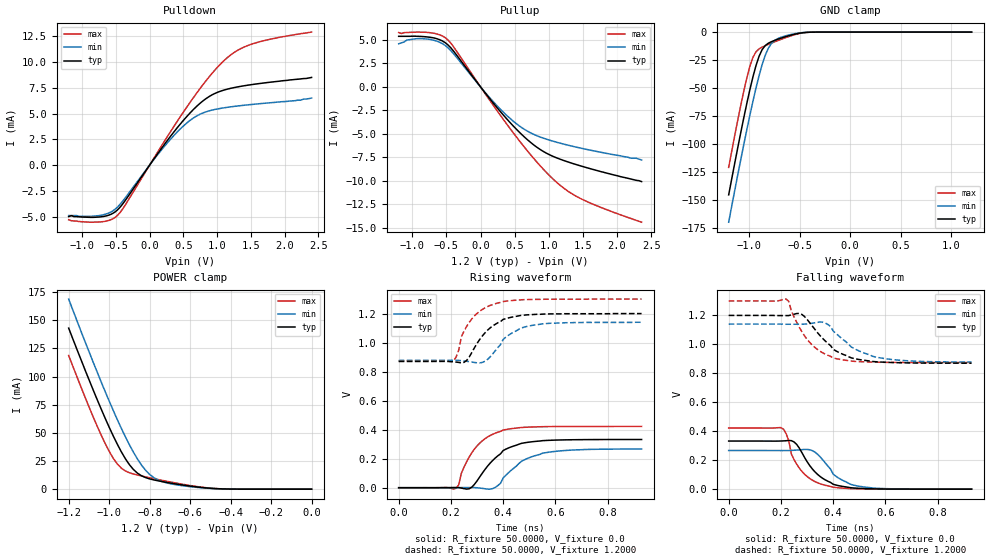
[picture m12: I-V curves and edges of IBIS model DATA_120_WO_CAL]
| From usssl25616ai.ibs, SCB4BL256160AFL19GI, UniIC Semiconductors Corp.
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|   Model DATA_120_WO_CAL
[Model]  DATA_120_WO_CAL
Model_type I/O
Polarity   Non-Inverting
Enable   Active-High
Vinl =   0.3800V
Vinh =   0.8200V
Vmeas =  0.6000V
Cref =   5.0000pF
Rref =   50.0000
Vref =   0.6000V
C_comp   1.7430pF   1.7110pF   1.7640pF
[Temperature Range]   25.0000   85.0000   -40.0000
[Voltage Range]   1.2000V   1.1400V   1.3000V
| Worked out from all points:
|   slope of the pulldown table from 0 to 0.18 V, typ, clamps not added: 108 ohm
|   slope of the pullup table from 0 to 0.18 V, typ, clamps not added: 108 ohm
|   GND clamp passes 1 mA (typ) near -0.50 V on its own axis
|   POWER clamp passes 1 mA (typ) near -0.51 V on its own axis
|   rising waveform, R_fixture 50.0000, V_fixture 0.0: 20-80 % time 103ps typ, 114ps min, 92.6ps max; typ from 0 V to 0.332 V
|   rising waveform, R_fixture 50.0000, V_fixture 1.2000: 20-80 % time 96ps typ, 92.4ps min, 78.1ps max; typ from 0.87 V to 1.2 V
|   falling waveform, R_fixture 50.0000, V_fixture 0.0: 20-80 % time 91.6ps typ, 90.4ps min, 73.1ps max; typ from 0.332 V to 0 V
|   falling waveform, R_fixture 50.0000, V_fixture 1.2000: 20-80 % time 115ps typ, 132ps min, 100ps max; typ from 1.2 V to 0.87 V
[Pulldown]
|Voltage   I(typ)   I(min)   I(max)
-1.2V     -5mA       -4.9mA     -5.3mA
-720mV    -5.02mA    -4.87mA    -5.507mA
-480mV    -4.371mA   -4.101mA   -4.906mA
-360mV    -3.417mA   -3.167mA   -3.855mA
200mV     1.839mA    1.668mA    2.116mA
520mV     4.485mA    3.908mA    5.332mA
680mV     5.593mA    4.698mA    6.829mA
840mV     6.469mA    5.177mA    8.219mA
1.2V      7.443mA    5.647mA    10.68mA
1.36V     7.649mA    5.774mA    11.33mA
1.6V      7.886mA    5.935mA    11.91mA
2.4V      8.5mA      6.5mA      12.9mA
[Pullup]
|Voltage   I(typ)   I(min)   I(max)
-1.2V     5.4mA      4.6mA      5.8mA
-1.08V    5.4mA      5mA        5.8mA
-880mV    5.39mA     5.16mA     5.84mA
-680mV    5.219mA    4.968mA    5.719mA
-520mV    4.73mA     4.433mA    5.263mA
-400mV    3.86mA     3.579mA    4.326mA
120mV     -1.12mA    -1.031mA   -1.272mA
440mV     -3.861mA   -3.41mA    -4.516mA
760mV     -6.076mA   -4.996mA   -7.465mA
1.08V     -7.464mA   -5.827mA   -9.945mA
1.48V     -8.455mA   -6.548mA   -11.96mA
2.36V     -10.1mA    -7.8mA     -14.43mA
[GND_clamp]
|Voltage   I(typ)   I(min)   I(max)
-1.2V     -145.3mA   -169.7mA   -120.8mA
-1.11V    -103.1mA   -127.3mA   -78.51mA
-1.05V    -76.2mA    -100.1mA   -52.43mA
-990mV    -51.2mA    -74mA      -30.39mA
-960mV    -39.9mA    -61.63mA   -22.48mA
-900mV    -21.67mA   -39mA      -15mA
-870mV    -15.78mA   -29.25mA   -13.45mA
-810mV    -10.04mA   -14.72mA   -11.07mA
-750mV    -7.557mA   -7.71mA    -8.865mA
-600mV    -3.111mA   -2.463mA   -3.804mA
-420mV    -215.4uA   -156.1uA   -235uA
1.2V      1.597nA    5.589nA    1.463nA
[POWER_clamp]
|Voltage   I(typ)   I(min)   I(max)
-1.2V     143mA      168.8mA    118.7mA
-1.06V    79.88mA    104.3mA    56.26mA
-1.02V    63.08mA    86.79mA    40.63mA
-980mV    47.32mA    69.97mA    27.48mA
-940mV    33.2mA     54.05mA    18.67mA
-880mV    17.43mA    32.78mA    13.45mA
-840mV    11.87mA    21.34mA    11.69mA
-800mV    9.133mA    13.1mA     10.12mA
-720mV    6.135mA    5.731mA    7.166mA
-560mV    1.838mA    1.456mA    2.161mA
-420mV    156.9uA    132.7uA    153uA
0V        1.597nA    1.927nA    2.16nA
[Ramp]
| variable   typ   min   max
dV/dt_r  0.1993/0.1052n   0.1601/0.1184n   0.2534/87.6937p
dV/dt_f  0.1979/0.1159n   0.1573/0.1322n   0.2551/93.0126p
R_load = 50.0000
[Rising Waveform]
R_fixture= 50.0000
V_fixture= 0.0
V_fixture_min= 0.0
V_fixture_max= 0.0
|time   V(typ)   V(min)   V(max)
0s        0V         0V         0V
220ps     1.212mV    191.5uV    -3.906mV
230ps     1.159mV    343uV      20.28mV
250ps     -6.397mV   813.1uV    141mV
290ps     22.9mV     785.4uV    266mV
360ps     188.1mV    -6.369mV   368.4mV
400ps     256.1mV    66.95mV    397.2mV
470ps     305.5mV    182mV      414.9mV
550ps     324.1mV    237.2mV    420.4mV
930ps     332.2mV    266.8mV    422.3mV
[Rising Waveform]
R_fixture= 50.0000
V_fixture= 1.2000
V_fixture_min= 1.1400
V_fixture_max= 1.3000
|time   V(typ)   V(min)   V(max)
0s        870mV      877.4mV    874.8mV
210ps     867.6mV    878mV      872.9mV
230ps     863.4mV    877.4mV    948.5mV
240ps     859.7mV    875.2mV    1.04V
280ps     931.8mV    866mV      1.163V
340ps     1.085V     883.7mV    1.248V
400ps     1.16V      1.022V     1.283V
470ps     1.188V     1.101V     1.295V
550ps     1.196V     1.129V     1.298V
930ps     1.2V       1.14V      1.3V
[Falling Waveform]
R_fixture= 50.0000
V_fixture= 0.0
V_fixture_min= 0.0
V_fixture_max= 0.0
|time   V(typ)   V(min)   V(max)
0s        332.3mV    267mV      422.3mV
210ps     333.4mV    266.6mV    414.3mV
230ps     336.1mV    266.8mV    334.8mV
240ps     335.1mV    267.9mV    242.5mV
270ps     284.7mV    271.2mV    146.3mV
320ps     140.3mV    266.4mV    62.41mV
370ps     63.8mV     180.8mV    26.57mV
420ps     24.55mV    77.69mV    9.531mV
500ps     5.841mV    20.03mV    2.048mV
930ps     3.658uV    18uV       748.3nV
[Falling Waveform]
R_fixture= 50.0000
V_fixture= 1.2000
V_fixture_min= 1.1400
V_fixture_max= 1.3000
|time   V(typ)   V(min)   V(max)
0s        1.2V       1.14V      1.3V
220ps     1.199V     1.139V     1.313V
230ps     1.199V     1.139V     1.297V
270ps     1.214V     1.139V     1.119V
300ps     1.173V     1.141V     1.035V
360ps     1.041V     1.153V     941.6mV
400ps     966.4mV    1.093V     906.5mV
470ps     906.6mV    981.5mV    884.4mV
560ps     880.6mV    913.9mV    876.9mV
930ps     870.1mV    877.9mV    874.8mV
